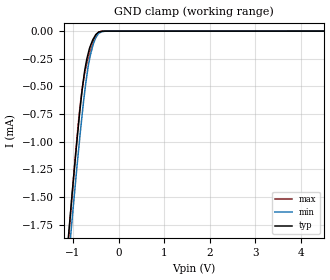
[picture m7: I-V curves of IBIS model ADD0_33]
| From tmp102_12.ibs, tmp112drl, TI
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|   ADD0_33   3.3V digital input Model
[Model] ADD0_33
Model_type   Input
| Signals   ADD0(4)
Vinl = 0.99
Vinh = 2.31
|   typ   min   max
|   (nom PVT)   (Fast PVT)   (slow PVT)
|Average
C_comp   5.4900270e-13  5.4418660e-13  5.5891410e-13
| Where   nom PVT is  Nominal Process, 3.3V, 27C
|   Fast PVT is Strong Process, 3.6V, -40C
|   Slow PVT is Weak Process, 3.0V, 125C
[Voltage Range]   3.3   3   3.6
[Temperature Range]   27   125   -40
|Ambient Temperature   27   125   -40
[Power Clamp Reference]   3.3   3   3.6
[GND Clamp Reference]   0   0   0
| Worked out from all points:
|   GND clamp passes 1 mA (typ) near -0.91 V on its own axis
[GND Clamp]
|   Voltage   I(typ)   I(min)   I(max)
-3.3V     -13.46mA   -13.1mA    -14.03mA
-1.087V   -1.801mA   -2.021mA   -1.829mA
-1.028V   -1.517mA   -1.747mA   -1.528mA
-938.5mV  -1.107mA   -1.342mA   -1.09mA
-840.7mV  -690.3uA   -922.9uA   -666.5uA
-746.4mV  -369.8uA   -564.8uA   -390.9uA
-669.3mV  -208.8uA   -328.8uA   -249.3uA
-622.2mV  -138.7uA   -224.4uA   -178.2uA
-550.1mV  -68.18uA   -112.6uA   -90.26uA
-431.8mV  -7.715uA   -20.4uA    -8.3uA
-283mV    -626.1nA   -693.1nA   -641.4nA
6.59V     0A         0A         0A
[POWER Clamp]
|   SCR cell for ESD function. Effects occurr above VDD x 2
|   Voltage   I(typ)   I(min)   I(max)
-3.3V     0A         0A         0A
0V        0A         0A         0A
6.6V      0A         0A         0A
